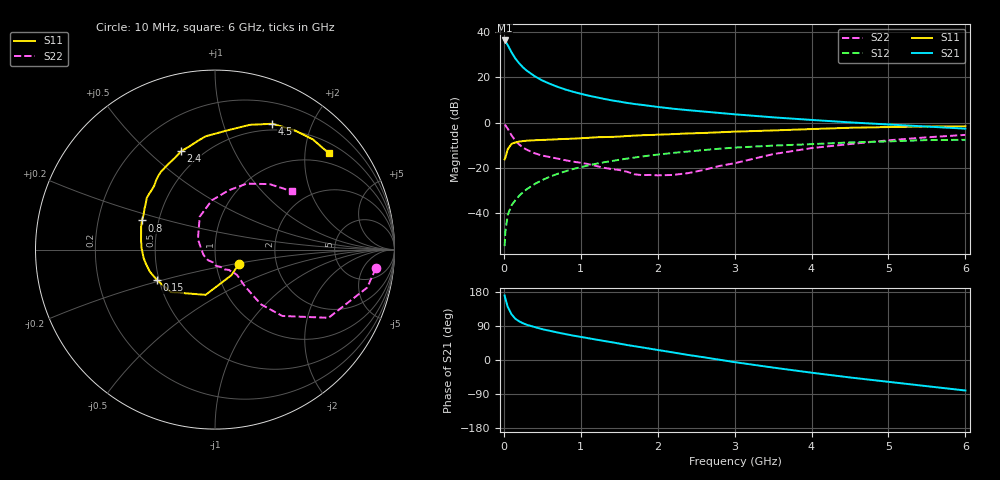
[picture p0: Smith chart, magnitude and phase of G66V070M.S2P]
! SIEMENS Small Signal Semiconductors
! BFG193
! Si NPN RF Bipolar Junction Transistor in SOT223
! VCE = 6 V  IC = 70 mA
! Common Emitter S-Parameters:  August  1996
# GHz  S  MA  R  50
!  f  S11  S21  S12  S22
! GHz  MAG  ANG  MAG  ANG  MAG  ANG  MAG  ANG
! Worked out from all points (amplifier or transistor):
!   36 points, 10 MHz to 6 GHz, reference 50 ohm
!   highest |S21| = 36.2 dB at 10 MHz (marker M1)
!   |S21| within 3 dB of that: start of sweep to 65.56 MHz
!   unconditionally stable (mu >= 1): 380.1 MHz to 2.38 GHz
!   at 250 MHz: K = 0.95, MSG = 27.5 dB, |S12| = -30.6 dB
!   at 1.4 GHz: K = 1.05, MAG = 12.1 dB, |S12| = -16.9 dB
!   at 6 GHz: K = 0.89, MSG = 2.5 dB, |S12| = -7.6 dB
!   S11 on the Smith chart (normalised r, x): 10 MHz: 1.29, -0.21; 150 MHz: 0.49, -0.19; 800 MHz: 0.40, +0.16; 2.4 GHz: 0.39, +0.64; 4.5 GHz: 0.43, +1.47; 6 GHz: 0.74, +2.55
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0.01  0.1554 -31.0  64.58 170.3  0.0019 84.5  0.9017 -6.7
0.02  0.1696 -57.4  61.73 162.1  0.004 83.7  0.874 -14.0
0.05  0.2575 -101.7  51.29 140.5  0.0092 71.7  0.7378 -31.0
0.1  0.3414 -136.1  35.44 120.5  0.0151 70.3  0.5267 -44.6
0.15  0.3654 -152.4  25.79 108.6  0.0196 68.7  0.3995 -49.9
0.2  0.3833 -161.3  20.2 102.0  0.0246 70.1  0.3305 -50.4
0.25  0.3928 -168.2  16.44 96.8  0.0294 70.3  0.2807 -50.6
0.3  0.4003 -173.2  13.9 92.8  0.0344 71.2  0.2525 -50.7
0.4  0.4094 178.9  10.56 87.0  0.0444 70.9  0.2117 -49.7
0.5  0.4157 172.4  8.48 81.3  0.0544 69.7  0.1879 -49.0
0.6  0.4218 167.4  7.134 76.9  0.0646 68.8  0.1741 -50.0
0.7  0.4309 162.7  6.134 72.5  0.0747 67.4  0.1613 -52.1
0.8  0.4379 158.2  5.362 68.4  0.0846 65.5  0.1482 -53.9
1.1  0.4624 146.7  3.935 57.4  0.1146 60.1  0.1219 -64.4
1.3  0.4806 140.1  3.342 50.3  0.1339 56.0  0.1012 -72.0
1.6  0.5076 130.1  2.725 39.6  0.1614 49.1  0.0829 -92.4
2.2  0.5584 113.4  2.026 19.9  0.2155 35.5  0.0704 -155.4
2.4  0.5791 109.1  1.878 13.2  0.2313 31.3  0.0774 176.7
3.5  0.6723 83.1  1.308 -20.0  0.3115 4.1  0.2022 114.9
4.5  0.7705 65.5  1.013 -46.1  0.3669 -15.9  0.3376 77.3
5.5  0.821 48.4  0.82 -69.1  0.4125 -39.4  0.4749 50.2
6  0.8313 40.1  0.737 -80.5  0.4186 -52.8  0.537 37.3
